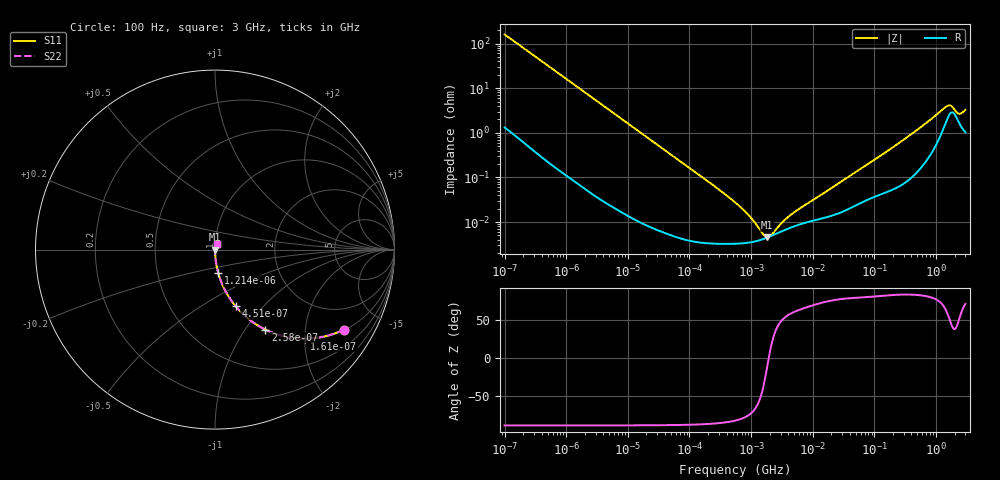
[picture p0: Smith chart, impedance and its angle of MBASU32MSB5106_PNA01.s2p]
! MBASU32MSB5106_PNA01  S-PARAMETER MODEL  ( Standard Model )
! Model Generated by TAIYO YUDEN Corporation (http://www.ty-top.com)
! Version 1.0
! TAIYO YUDEN Control No. 220601
! Copyright(c) 2015 TAIYO YUDEN CO.,LTD. All Rights Reserved.
! Product Description (link to TY-COMPAS)
! https://ds.yuden.co.jp/TYCOMPAS/or/detail?pn=MBASU32MSB5106KPNA01&u=M
! Products Name : Multilayer Ceramic Capacitors
! Characteristics :
!  Capacitance : 10 [uF] , Rated Voltage : 50 [V] , TCC : X5R
!  Case Size : 3.2 x 2.5 / 0.126 x 0.098 [mm/inch] , Thickness : 2.5 / 0.098 [mm/inch]
!  (Conditions: Temperature = 25 [degC] , DC Bias Voltage = 0 [V])
! External Node Assignments :
!  1  o---| |---o  2
! GND o---------o GND
! Frequency Range : 100Hz  -  3GHz  [ 401 STEP ]
# MHZ S RI R 50
! Freq[MHz].  S11 Real  S11 Imag  S21 Real  S21 Imag  S12 Real  S12 Imag  S22 Real  S22 Imag
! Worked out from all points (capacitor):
!   401 points, 100 Hz to 3 GHz, reference 50 ohm
!   read as one part in series: C = 9.95 uF near 109 Hz
!   lowest |Z| = 4.58 mohm at 1.828 MHz (marker M1)
!   series resonance near 1.933 MHz, so ESL is about 680 pH
!   S11 on the Smith chart (normalised r, x): 100 Hz: 1.03, -3.19; 161 Hz: 1.02, -1.99; 258 Hz: 1.01, -1.25; 451 Hz: 1.00, -0.71; 1.214 kHz: 1.00, -0.27; 3 GHz: 1.02, +0.06
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0.0001  0.7167 -0.4465  0.2833 0.4465  0.2833 0.4465  0.7167 -0.4465
0.000161  0.4987 -0.4961  0.5013 0.4961  0.5013 0.4961  0.4987 -0.4961
0.000258  0.2809 -0.4457  0.7191 0.4457  0.7191 0.4457  0.2809 -0.4457
0.000451  0.1146 -0.3151  0.8854 0.3151  0.8854 0.3151  0.1146 -0.3151
0.000694  0.0526 -0.2198  0.9474 0.2198  0.9474 0.2198  0.0526 -0.2198
0.001214  0.0183 -0.1305  0.9817 0.1305  0.9817 0.1305  0.0183 -0.1305
0.001788  0.00872 -0.0896  0.9913 0.0896  0.9913 0.0896  0.00872 -0.0896
0.005476  0.0011 -0.0296  0.9989 0.0296  0.9989 0.0296  0.0011 -0.0296
0.031977  9.01e-05 -0.00512  0.9999 0.00512  0.9999 0.00512  9.01e-05 -0.00512
0.221826  3.36e-05 -0.000733  1 0.000733  1 0.000733  3.36e-05 -0.000733
0.547723  3.27e-05 -0.000275  1 0.000275  1 0.000275  3.27e-05 -0.000275
1.138514  3.66e-05 -9.21e-05  1 9.21e-05  1 9.21e-05  3.66e-05 -9.21e-05
1.827928  4.49e-05 -8.85e-06  1 8.85e-06  1 8.85e-06  4.49e-05 -8.85e-06
3.198641  6.27e-05 7.59e-05  0.9999 -7.59e-05  0.9999 -7.59e-05  6.27e-05 7.59e-05
9.794414  0.000106 0.000285  0.9999 -0.000285  0.9999 -0.000285  0.000106 0.000285
175.1444  0.00051 0.00414  0.9995 -0.00414  0.9995 -0.00414  0.00051 0.00414
536.3016  0.00164 0.0125  0.9984 -0.0125  0.9984 -0.0125  0.00164 0.0125
1506.733  0.0203 0.0331  0.9797 -0.0331  0.9797 -0.0331  0.0203 0.0331
1789.813  0.0286 0.0259  0.9714 -0.0259  0.9714 -0.0259  0.0286 0.0259
2317.205  0.0178 0.0194  0.9822 -0.0194  0.9822 -0.0194  0.0178 0.0194
2525.516  0.0145 0.0224  0.9855 -0.0224  0.9855 -0.0224  0.0145 0.0224
3000  0.0112 0.0304  0.9888 -0.0304  0.9888 -0.0304  0.0112 0.0304
